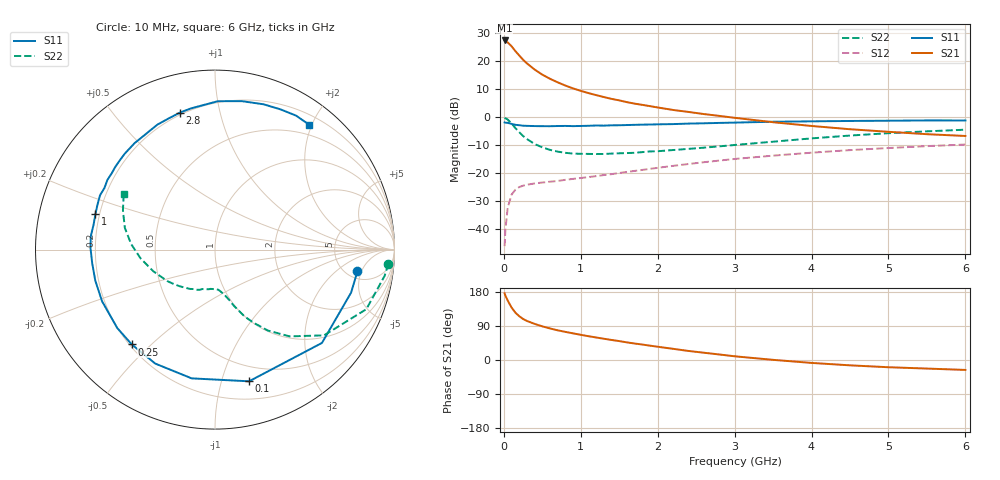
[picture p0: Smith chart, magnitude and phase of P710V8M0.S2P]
! SIEMENS Small Signal Semiconductors
! BFP196
! Si NPN RF Bipolar Junction Transistor in SOT143
! VCE = 10 V  IC = 8 mA
! Common Emitter S-Parameters:  May  1996
# GHz  S  MA  R  50
!  f  S11  S21  S12  S22
! GHz  MAG  ANG  MAG  ANG  MAG  ANG  MAG  ANG
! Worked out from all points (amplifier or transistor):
!   36 points, 10 MHz to 6 GHz, reference 50 ohm
!   highest |S21| = 27.3 dB at 10 MHz (marker M1)
!   |S21| within 3 dB of that: start of sweep to 127 MHz
!   unconditionally stable (mu >= 1): 999.4 MHz to 3.291 GHz
!   at 250 MHz: K = 0.33, MSG = 22.5 dB, |S12| = -24.5 dB
!   at 1.4 GHz: K = 1.13, MAG = 11.2 dB, |S12| = -20.3 dB
!   at 6 GHz: K = 0.97, MSG = 1.5 dB, |S12| = -9.8 dB
!   S11 on the Smith chart (normalised r, x): 10 MHz: 6.24, -4.22; 100 MHz: 0.36, -1.23; 250 MHz: 0.21, -0.44; 1 GHz: 0.18, +0.14; 2.8 GHz: 0.19, +0.76; 6 GHz: 0.34, +1.95
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0.01  0.8029 -8.6  23.26 175.9  0.005 83.9  0.9698 -4.7
0.02  0.7953 -17.5  22.68 170.0  0.0098 79.0  0.9558 -8.9
0.05  0.7909 -41.1  21.46 157.0  0.0241 69.0  0.9061 -21.5
0.1  0.7579 -75.5  18.36 138.6  0.0414 54.7  0.7727 -38.2
0.15  0.7291 -100.3  15.01 124.9  0.0507 44.6  0.6377 -49.3
0.2  0.717 -117.7  12.56 115.6  0.0566 38.5  0.5392 -56.8
0.25  0.703 -131.3  10.54 108.3  0.0599 34.7  0.4605 -62.2
0.3  0.6983 -141.2  9.077 103.1  0.0623 32.4  0.4067 -66.2
0.4  0.692 -155.4  7.046 95.3  0.0657 29.6  0.3315 -71.3
0.5  0.689 -165.5  5.709 88.8  0.0682 29.5  0.2886 -74.5
0.6  0.6884 -173.7  4.826 83.3  0.0705 30.2  0.2606 -77.8
0.7  0.6936 179.4  4.165 78.3  0.0727 31.2  0.2426 -80.9
0.8  0.6963 174.0  3.652 74.2  0.0762 32.0  0.2309 -83.4
1  0.6949 163.5  2.938 66.5  0.0821 34.5  0.2218 -87.7
1.1  0.7006 159.3  2.682 62.8  0.0853 35.4  0.2207 -90.7
1.6  0.722 140.2  1.848 46.5  0.1053 39.7  0.2286 -105.3
2.2  0.7504 120.9  1.341 29.5  0.1351 40.4  0.2589 -122.2
2.8  0.7879 104.3  1.052 14.6  0.1678 37.6  0.3008 -140.7
3.5  0.8269 88.9  0.811 0.4  0.2056 31.4  0.3645 -160.7
4.5  0.8535 71.6  0.608 -14.1  0.258 21.2  0.469 176.1
5.5  0.8725 58.8  0.496 -22.6  0.3036 9.8  0.5577 156.9
6  0.8714 53.1  0.461 -26.2  0.3245 3.6  0.5966 148.5
